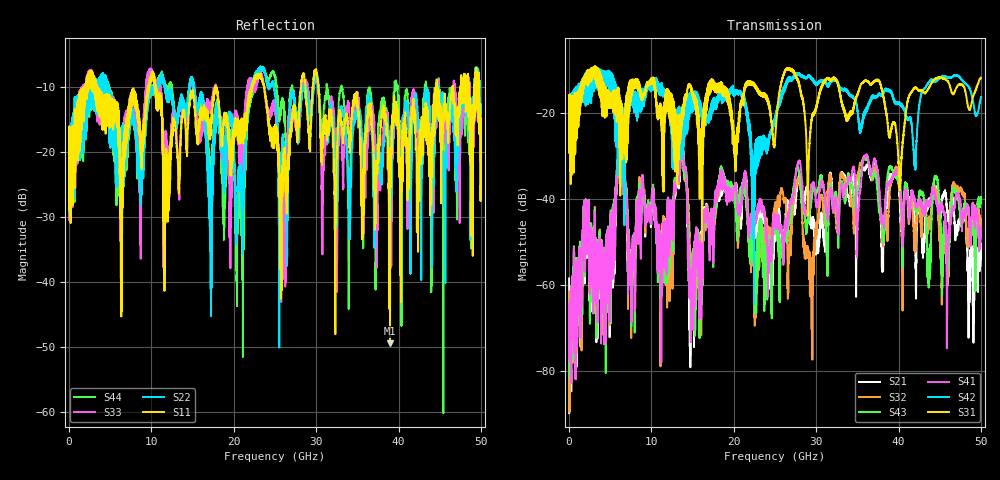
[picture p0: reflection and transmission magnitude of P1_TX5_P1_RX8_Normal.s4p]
!Keysight Technologies,N5225B,MY57041031,A.13.20.10
!Date: Friday, May 31, 2019 11:26:02
!Correction: S11(Full 4 Port(1,2,3,4))
!S12(Full 4 Port(1,2,3,4))
!S13(Full 4 Port(1,2,3,4))
!S14(Full 4 Port(1,2,3,4))
!S21(Full 4 Port(1,2,3,4))
!S22(Full 4 Port(1,2,3,4))
!S23(Full 4 Port(1,2,3,4))
!S24(Full 4 Port(1,2,3,4))
!S31(Full 4 Port(1,2,3,4))
!S32(Full 4 Port(1,2,3,4))
!S33(Full 4 Port(1,2,3,4))
!S34(Full 4 Port(1,2,3,4))
!S41(Full 4 Port(1,2,3,4))
!S42(Full 4 Port(1,2,3,4))
!S43(Full 4 Port(1,2,3,4))
!S44(Full 4 Port(1,2,3,4))
!S4P File: Measurements: <S11,S12,S13,S14>,
!<S21,S22,S23,S24>,
!<S31,S32,S33,S34>,
!<S41,S42,S43,S44>:
# Hz S  dB  R 50.0
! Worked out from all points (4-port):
!   5000 points, 10 MHz to 50 GHz, reference 50 ohm
!   strongest paths, dB at 10 MHz, 12.51 GHz, 25.01 GHz, 37.51 GHz, 50 GHz:
!     S31: -19.6, -23.0, -26.1, -12.3, -11.7
!     S42: -19.5, -24.2, -21.8, -15.9, -16.2
!     S41: -68.9, -48.3, -45.8, -34.5, -46.7
!     S43: -68.4, -49.9, -45.2, -39.6, -39.5
!     S32: -61.5, -58.7, -43.1, -36.0, -45.4
!     S21: -58.4, -51.8, -48.9, -34.4, -50.7
!   lowest |S11| = -49.4 dB at 38.97 GHz (marker M1), VSWR 1.01, Z = 50 - j0.337 ohm
!   |S11| at or under -10 dB: 3.363 GHz to 9.558 GHz (6.195 GHz wide, 95.9 % of centre); 10.5 GHz to 17.75 GHz (7.242 GHz wide, 51.3 % of centre); 30.28 GHz to 44.61 GHz (14.33 GHz wide, 38.3 % of centre)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
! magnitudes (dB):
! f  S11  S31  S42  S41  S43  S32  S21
! 10 MHz  -19.3  -19.6  -19.5  -68.9  -68.4  -61.5  -58.4
! 6.18 GHz  -20.2  -29.6  -20.4  -27.9  -27.4  -27.8  -28.5
! 7.57 GHz  -12.6  -13.9  -17.2  -59.7  -59.6  -56.5  -56.8
! 13.78 GHz  -14.2  -19.2  -19.8  -28.4  -29.0  -28.3  -28.0
! 14.83 GHz  -11.1  -14.6  -16.7  -66.6  -63.0  -61.0  -59.4
! 38.97 GHz  -49.4  -25.1  -14.8  -36.2  -32.4  -37.3  -34.6
! 50 GHz  -14.8  -11.7  -16.2  -46.7  -39.5  -45.4  -50.7
